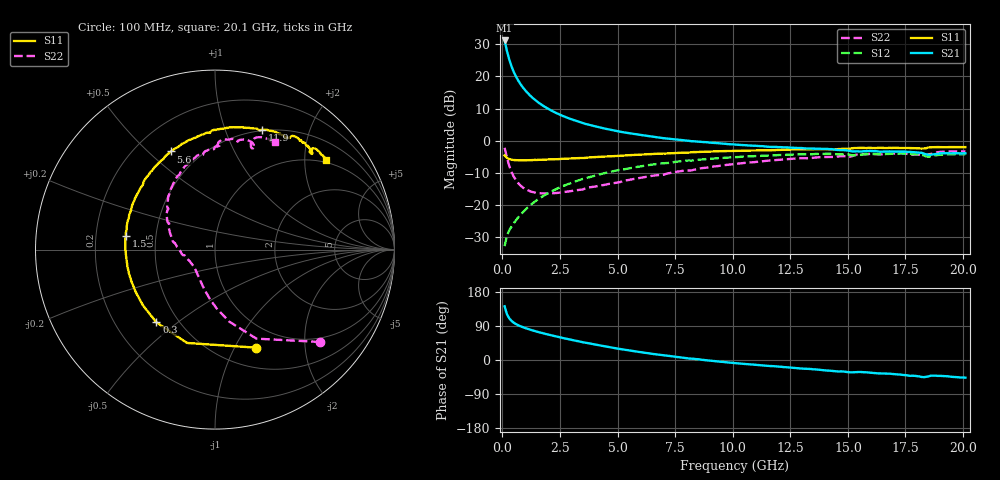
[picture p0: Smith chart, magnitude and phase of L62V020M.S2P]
!  Infineon Technologies AG
! BFR380L3 , PF131585-7, No.6, Th 09.10.01, soldered on pcb-board, measured with PP GSG850
!  Vce=2.0 V,  Ic=20.0 mA
! Common Emitter S-Parameters:  15. November 2001
#  GHz  S  MA  R  50
! f  S11  S21  S12  S22
! GHz  Mag  Ang  Mag  Ang  Mag  Ang  Mag  Ang
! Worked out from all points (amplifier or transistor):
!   201 points, 100 MHz to 20.1 GHz, reference 50 ohm
!   highest |S21| = 31.2 dB at 100 MHz (marker M1)
!   |S21| within 3 dB of that: start of sweep to 193.3 MHz
!   unconditionally stable (mu >= 1): 1.396 GHz to 4.474 GHz
!   at 3.4 GHz: K = 1.02, MAG = 8.1 dB, |S12| = -12.1 dB
!   at 10.1 GHz: K = 0.96, MSG = 2.0 dB, |S12| = -5.1 dB
!   at 20.1 GHz: K = 0.99, MSG = 0.1 dB, |S12| = -4.2 dB
!   S11 on the Smith chart (normalised r, x): 100 MHz: 0.73, -1.22; 300 MHz: 0.38, -0.42; 1.5 GHz: 0.33, +0.07; 5.6 GHz: 0.35, +0.59; 11.9 GHz: 0.49, +1.35; 20.1 GHz: 0.93, +2.53
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0.1  0.5918 -67.4  36.3 141.8  0.02293 65.1  0.7784 -41.4
0.2  0.543 -106.7  25.07 121.0  0.03315 54.4  0.547 -65.1
0.3  0.5205 -128.9  18.39 110.1  0.04041 53.6  0.4088 -78.8
0.4  0.5077 -142.2  14.35 103.2  0.04625 54.5  0.3271 -88.5
0.5  0.5011 -151.6  11.7 98.2  0.05218 56.5  0.2759 -96.0
0.6  0.4983 -158.6  9.866 94.6  0.0584 58.2  0.2415 -102.3
0.7  0.4975 -164.2  8.533 91.5  0.06484 59.6  0.2172 -107.8
0.8  0.497 -168.6  7.504 88.7  0.07144 60.8  0.1996 -112.6
1  0.4968 -175.7  6.059 84.1  0.08471 62.4  0.177 -120.8
1.2  0.5001 178.7  5.081 80.2  0.09838 63.2  0.1643 -127.7
1.5  0.5025 171.4  4.105 74.9  0.1191 63.5  0.1543 -136.3
1.8  0.508 165.5  3.448 70.0  0.14 63.0  0.151 -143.4
2.3  0.5157 156.6  2.744 62.6  0.1744 61.2  0.1537 -153.3
2.9  0.5298 147.2  2.223 54.5  0.2151 58.1  0.1633 -162.8
3.5  0.5396 138.5  1.88 46.8  0.2551 54.4  0.1747 -169.8
5.6  0.5996 114.2  1.297 24.5  0.3781 40.4  0.2505 164.6
6.8  0.6278 102.4  1.123 13.7  0.4394 31.9  0.2931 151.1
10.1  0.6975 77.9  0.8725 -8.2  0.556 10.5  0.4356 122.2
11.9  0.7173 68.7  0.802 -17.0  0.5965 -0.0  0.5003 107.5
13.5  0.7362 60.6  0.7565 -24.6  0.6186 -9.8  0.5448 96.4
16.8  0.7756 48.4  0.6826 -36.1  0.6247 -25.5  0.6304 76.3
20.1  0.7957 38.9  0.6396 -46.7  0.6185 -38.9  0.6849 60.6
